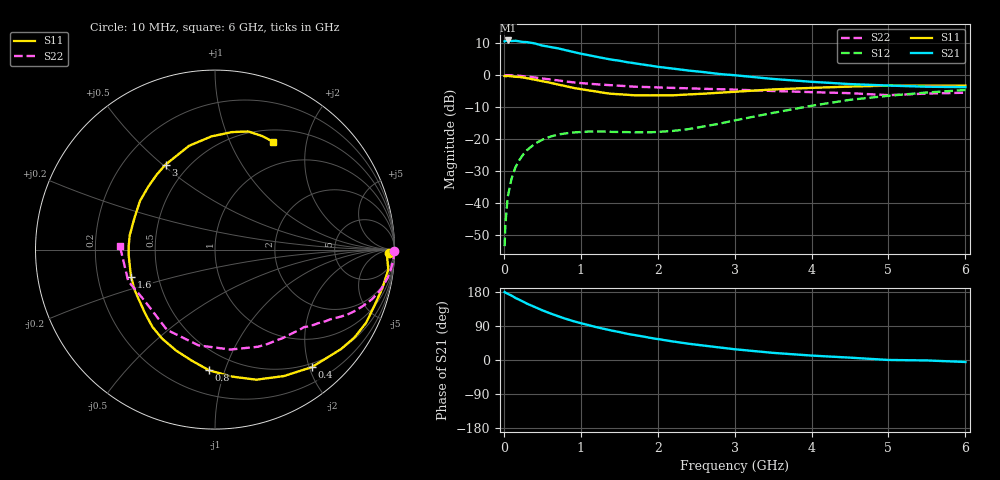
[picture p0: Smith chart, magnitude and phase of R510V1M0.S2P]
! SIEMENS Small Signal Semiconductors
! BFR183
! Si NPN RF Bipolar Junction Transistor in SOT23
! VCE = 10 V  IC = 1 mA
! Common Emitter S-Parameters:  May  1996
# GHz  S  MA  R  50
!  f  S11  S21  S12  S22
! GHz  MAG  ANG  MAG  ANG  MAG  ANG  MAG  ANG
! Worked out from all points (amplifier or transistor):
!   36 points, 10 MHz to 6 GHz, reference 50 ohm
!   highest |S21| = 10.8 dB at 50 MHz (marker M1)
!   |S21| within 3 dB of that: start of sweep to 797.2 MHz
!   unconditionally stable (mu >= 1): 1.688 GHz to 2.977 GHz
!   at 250 MHz: K = 0.15, MSG = 17.6 dB, |S12| = -24.9 dB
!   at 1.4 GHz: K = 0.83, MSG = 11.3 dB, |S12| = -17.8 dB
!   at 6 GHz: K = 0.94, MSG = 0.4 dB, |S12| = -4.7 dB
!   S11 on the Smith chart (normalised r, x): 10 MHz: 43, -27; 400 MHz: 0.44, -2.04; 800 MHz: 0.36, -0.89; 1.6 GHz: 0.35, -0.14; 3 GHz: 0.38, +0.51; 6 GHz: 0.65, +1.47
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0.01  0.9672 -1.2  3.38 179.3  0.0021 88.5  0.9975 -0.4
0.02  0.9599 -2.5  3.43 177.8  0.0046 84.2  0.9921 -0.9
0.05  0.9721 -6.6  3.484 174.8  0.0123 84.2  0.9968 -2.5
0.1  0.9569 -13.0  3.412 170.0  0.0239 81.8  0.9908 -4.8
0.15  0.9411 -19.7  3.444 163.9  0.0358 77.9  0.9836 -7.2
0.3  0.8945 -38.3  3.283 148.7  0.0667 67.3  0.9496 -13.6
0.4  0.8486 -50.5  3.139 140.1  0.0837 60.3  0.918 -17.5
0.5  0.8024 -61.4  2.897 131.1  0.0973 54.7  0.8847 -20.6
0.6  0.7604 -72.4  2.76 123.3  0.1084 49.7  0.8558 -23.3
0.7  0.7126 -82.7  2.627 115.9  0.1172 45.3  0.8269 -25.7
0.8  0.6734 -92.8  2.462 109.0  0.1221 41.5  0.7964 -27.9
0.9  0.6315 -102.0  2.308 102.8  0.1264 38.7  0.7704 -29.7
1.1  0.5767 -120.8  2.052 92.1  0.1306 34.3  0.7343 -32.9
1.3  0.5277 -137.4  1.839 82.3  0.1309 31.7  0.705 -35.6
1.6  0.492 -161.9  1.594 69.3  0.1281 32.3  0.6711 -39.7
1.9  0.4812 177.4  1.41 58.6  0.1273 37.4  0.6481 -44.1
2.2  0.4824 158.3  1.263 48.9  0.1339 44.1  0.6301 -48.8
3  0.5478 120.2  0.995 28.4  0.1951 57.0  0.5917 -66.2
3.5  0.5962 104.0  0.87 18.8  0.2563 56.6  0.5635 -81.2
4.5  0.6611 81.9  0.723 6.2  0.4104 45.0  0.5213 -120.9
5.5  0.6852 67.2  0.657 -1.2  0.5339 28.1  0.5143 -160.0
6  0.6821 61.6  0.648 -5.2  0.5845 18.0  0.5298 178.1
